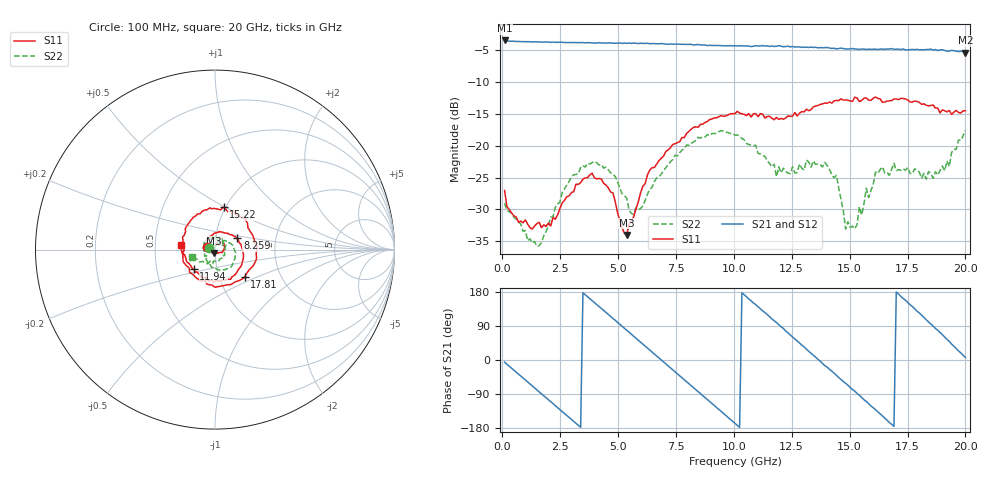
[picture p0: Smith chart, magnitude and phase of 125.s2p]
!Agilent Technologies,N5230C,MY49001569,A.09.33.09
!Agilent N5230C: A.09.33.09
!Date: Tuesday, July 28, 2015 18:44:44
!Correction: S11(Full 2 Port(1,2))
!S21(Full 2 Port(1,2))
!S12(Full 2 Port(1,2))
!S22(Full 2 Port(1,2))
!S2P File: Measurements: S11, S21, S12, S22:
# Hz S  dB  R 50
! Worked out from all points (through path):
!   201 points, 100 MHz to 20 GHz, reference 50 ohm
!   highest |S21| = -3.43 dB at 100 MHz (marker M1); lowest = -5.3 dB at 20 GHz (marker M2)
!   group delay of S21, straight-line fit = 148 ps
!   lowest |S11| = -34.0 dB at 5.373 GHz (marker M3), VSWR 1.04, Z = 49.2 - j1.79 ohm
!   |S11| at or under -10 dB: start of sweep to end of sweep
!   |S22| runs from -35.8 to -17.6 dB; largest |S21 - S12| = 0.024
!   S11 on the Smith chart (normalised r, x): 100 MHz: 0.92, +0.03; 8.259 GHz: 1.27, +0.16; 11.94 GHz: 0.77, -0.17; 15.22 GHz: 0.98, +0.49; 17.81 GHz: 1.32, -0.42; 20 GHz: 0.68, +0.03
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1e8  -27.01 161.8  -3.43 -5.8  -3.44 -5.7  -29.02 161.3
6.97e8  -31.99 115.3  -3.59 -37.2  -3.60 -37.2  -31.96 132.4
1.7915e9  -32.43 81.5  -3.71 -94.6  -3.68 -94.2  -34.12 131.6
3.483e9  -25.21 48.5  -3.76 177.5  -3.79 177.3  -23.11 89.5
4.7765e9  -27.38 -23.1  -3.86 109.7  -3.87 109.9  -24.44 41.5
5.3735e9  -34.00 -114.2  -3.89 78.8  -3.85 78.3  -28.22 34.2
5.672e9  -31.20 -155.0  -3.83 62.7  -3.90 62.9  -30.77 47.6
6.7665e9  -22.32 114.7  -3.96 5.3  -3.90 5.4  -24.89 57.3
8.259e9  -17.09 26.8  -4.13 -73.1  -4.12 -73.2  -19.37 0.1
9.055e9  -15.77 -13.7  -4.22 -114.9  -4.22 -114.8  -18.06 -30.5
1.005e10  -14.94 -58.2  -4.27 -167.1  -4.34 -166.9  -18.31 -68.4
1.0846e10  -14.96 -89.1  -4.33 150.3  -4.30 151.4  -19.97 -97.6
1.19405e10  -15.84 -137.1  -4.25 93.6  -4.33 92.4  -23.30 -146.9
1.3433e10  -13.87 145.1  -4.53 12.6  -4.55 12.4  -22.38 117.4
1.4428e10  -12.86 104.4  -4.76 -40.2  -4.65 -40.0  -24.64 76.8
1.4826e10  -12.78 92.3  -4.79 -61.5  -4.75 -62.2  -33.08 80.8
1.5224e10  -12.35 78.6  -4.76 -82.5  -4.77 -84.0  -33.05 127.8
1.61195e10  -12.33 44.3  -4.80 -131.3  -4.77 -131.4  -24.13 121.9
1.67165e10  -12.93 15.1  -4.78 -164.9  -4.79 -164.7  -24.64 97.6
1.7811e10  -12.96 -42.9  -4.88 135.0  -4.83 135.3  -23.62 28.4
1.8806e10  -14.06 -102.9  -5.02 78.5  -4.87 78.2  -24.60 -65.4
2e10  -14.48 172.9  -5.33 6.5  -5.45 6.5  -17.56 -161.6
